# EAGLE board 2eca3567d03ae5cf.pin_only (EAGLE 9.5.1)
REV: B

Size 25.4 x 17.78 mm. Coordinates in mm from the lower left corner, seen from the top.
Outline: 0,15.24 0,2.54 arc90 2.54,0 22.86,0 arc90 25.4,2.54 25.4,15.24 arc90 22.86,17.78 2.54,17.78 arc90 0,15.24
Copper layers (1*16): Top 0.035mm / dielectric 1.5mm / Bottom 0.035mm
Design rules "adafruit 7-7": minimum track width 6mil, minimum drill 15.5mil, track to track 8mil, track to pad 7mil, pad to pad 7mil, via to via 7mil, smd to smd 7mil, copper to edge 10mil, drill to drill 8mil, minimum pad ring 10mil, minimum via ring 8mil, stop-mask expansion 2mil, vias tented up to drill 20mil, thermal gap 10mil
Net classes: 1 highpower: width 0.406 mm, drill 0.483 mm; 2 lowpower: width 0.305 mm, drill 0.483 mm

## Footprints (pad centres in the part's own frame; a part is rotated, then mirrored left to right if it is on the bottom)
0603-NO = smd 1.075 x 1: 1 -0.85,0; 2 0.85,0
0805-NO = smd 1.24 x 1.5: 1 -0.95,0; 2 0.95,0
JST_SH4 = smd 0.6 x 1.55: 1 -1.5,2.514; 2 -0.5,2.514; 3 0.5,2.514; 4 1.5,2.514 | smd 1.2 x 1.8: MT1 -2.8,-1.386; MT2 2.8,-1.386
CHIPLED_0603_NOOUTLINE = smd 0.8 x 0.8: A 0,-0.75; C 0,0.75
FIDUCIAL_1MM = smd 1 x 1: 1 0,0
1X06_ROUND = drill 1 pad 1.676: 1 -6.35,0; 2 -3.81,0; 3 -1.27,0; 4 1.27,0; 5 3.81,0; 6 6.35,0
1X06_ROUND_70 = drill 1 pad 1.778: 1 -6.35,0; 2 -3.81,0; 3 -1.27,0; 4 1.27,0; 5 3.81,0; 6 6.35,0
SOT363 = smd 0.5 x 0.5: 1 -0.75,-0.9; 3 0.75,-0.9; 4 0.75,0.9; 6 -0.75,0.9 | smd 0.4 x 0.5: 2 0,-0.9; 5 0,0.9
RESPACK_4X0603 = smd 0.45 x 0.9: 1 -1.3,-0.85; 2 -0.4,-0.85; 3 0.4,-0.85; 4 1.3,-0.85; 5 1.3,0.85; 6 0.4,0.85; 7 -0.4,0.85; 8 -1.3,0.85
SOLDERJUMPER_CLOSEDWIRE = smd 1.168 x 1.6: 1 -0.762,0; 2 0.762,0 | smd 0.635 x 0.203: WIRE 0,0
SOLDERJUMPER_ARROW_NOPASTE = smd 0.762 x 1.524: 1 -1.016,0; 2 1.016,0
QFN24_4MM_SMSC = smd 0.8 x 0.28: 1 -2,1.25; 2 -2,0.75; 3 -2,0.25; 4 -2,-0.25; 5 -2,-0.75; 6 -2,-1.25; 13 2,-1.25; 14 2,-0.75; 15 2,-0.25; 16 2,0.25; 17 2,0.75; 18 2,1.25 | smd 0.28 x 0.8: 7 -1.25,-2; 8 -0.75,-2; 9 -0.25,-2; 10 0.25,-2; 11 0.75,-2; 12 1.25,-2; 19 1.25,2; 20 0.75,2; 21 0.25,2; 22 -0.25,2; 23 -0.75,2; 24 -1.25,2 | smd 2.5 x 2.5: THERM 0,0
SOT23-5 = smd 0.55 x 1.2: 1 -0.95,-1.3; 2 0,-1.3; 3 0.95,-1.3; 4 0.95,1.3; 5 -0.95,1.3
MOUNTINGHOLE_2.5_PLATED = drill 2.5 pad 3.2: P$1 0,0

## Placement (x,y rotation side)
C1  2.2nF  [0603-NO]  16.05,6.1 270 top
C2  0.1uF  [0603-NO]  9.73,5.47 270 top
C5  10uF  [0805-NO]  7.34,4.93 0 top
C6  10uF  [0805-NO]  7.05,11.54 90 top
C7  0.1uF  [0603-NO]  13.45,5.59 0 top
CONN3  STEMMA_I2C_QT  [JST_SH4]  22.86,8.89 90 top
CONN4  STEMMA_I2C_QT  [JST_SH4]  2.54,8.89 270 top
D1  GREEN  [CHIPLED_0603_NOOUTLINE]  3.56,12.57 90 top
FID3  FIDUCIAL_1MM  [FIDUCIAL_1MM]  20.07,13.14 0 top
FID4  FIDUCIAL_1MM  [FIDUCIAL_1MM]  4.66,4.75 0 top
JP2  [1X06_ROUND]  12.7,15.24 0 top
JP3  [1X06_ROUND_70]  12.7,2.54 0 top
Q2  BSS138  [SOT363]  18.31,6.15 180 top
R2  10K  [0603-NO]  8.93,11.63 90 top
R3  10K  [RESPACK_4X0603]  17.42,10.54 180 top
R4  10K  [0603-NO]  5.47,12.41 90 top
SJ1  CLKIN  [SOLDERJUMPER_CLOSEDWIRE]  16.13,11.81 180 bottom
SJ2  FSYNC  [SOLDERJUMPER_CLOSEDWIRE]  12.06,11.81 0 bottom
SJ3  [SOLDERJUMPER_ARROW_NOPASTE]  6.6,11.81 0 bottom
U1  MPU-6050  [QFN24_4MM_SMSC]  12.7,8.89 270 top
U3  AP2112K-3.3  [SOT23-5]  7.7,7.87 0 top
U$39  MOUNTINGHOLE2.5  [MOUNTINGHOLE_2.5_PLATED]  2.54,15.24 0 top
U$40  MOUNTINGHOLE2.5  [MOUNTINGHOLE_2.5_PLATED]  22.86,15.24 0 top
U$42  MOUNTINGHOLE2.5  [MOUNTINGHOLE_2.5_PLATED]  2.54,2.54 0 top
U$43  MOUNTINGHOLE2.5  [MOUNTINGHOLE_2.5_PLATED]  22.86,2.54 0 top
U$46  [PCBFEAT-REV-040]  20.32,13.46 0 bottom
U$47  [STEMMAQT]  22.48,4.45 90 bottom
U$48  [STEMMAQT]  2.92,13.34 270 bottom

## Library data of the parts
C1 C2 C5-C7 CONN3 CONN4 D1 JP2 JP3 Q2 R2-R4 SJ1 SJ2 U1 U3 U$46 = microbuilder
FID3 FID4 SJ3 U$39 U$40 U$42 U$43 = microbuilder; BOM: EXCLUDE
U$47 U$48 = silks

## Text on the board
tPlace: MPU-6050 6-DoF | on | X | Y | Z | SCL | INT | VIN | 3Vo | GND | SDA
bPlace: FS | SCE | SDE | GND | AD0 | FSYNC | CLKIN | 6DoF Accel/Gyro | Gyro ±250~2000 dps | Accel ±2/4/8/16 g | Default I2C Addr 0x68 | I2C Logic/Vcc: 3-5VDC

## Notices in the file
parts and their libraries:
microbuilder: This work is placed in the public domain, and may be freely used for commercial and non-commercial work with the following conditions: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
